FUNCTION_BLOCK FB_LN_IED_LD1_ATCC1 EXTENDS FB_AcsiCommonLogicalNodeClass
VAR_INPUT
	NamPlt: FB_DO_IED_LD1_ATCC1_NamPlt := (sClass:='LPL', bLinkResult:=THIS^.AddDataToContainer(ipData:=NamPlt));
	Beh: FB_DO_IED_LD1_ATCC1_Beh := (sClass:='ENS', bLinkResult:=THIS^.AddDataToContainer(ipData:=Beh));
	Mod_: FB_DO_IED_LD1_ATCC1_Mod := (sObjectName:='Mod', sClass:='ENC', bLinkResult:=THIS^.AddDataToContainer(ipData:=Mod_));
	LocKey: FB_DO_IED_LD1_ATCC1_LocKey := (sClass:='SPS', bLinkResult:=THIS^.AddDataToContainer(ipData:=LocKey));
	CtlV: FB_DO_IED_LD1_ATCC1_CtlV := (sClass:='MV', bLinkResult:=THIS^.AddDataToContainer(ipData:=CtlV));
	TapChg: FB_DO_IED_LD1_ATCC1_TapChg := (sClass:='BSC', bLinkResult:=THIS^.AddDataToContainer(ipData:=TapChg));
	TapPos: FB_DO_IED_LD1_ATCC1_TapPos := (sClass:='ISC', bLinkResult:=THIS^.AddDataToContainer(ipData:=TapPos));
	BndCtrChg: FB_DO_IED_LD1_ATCC1_BndCtrChg := (sClass:='BAC', bLinkResult:=THIS^.AddDataToContainer(ipData:=BndCtrChg));
	ParOp: FB_DO_IED_LD1_ATCC1_ParOp := (sClass:='SPC', bLinkResult:=THIS^.AddDataToContainer(ipData:=ParOp));
END_VAR
VAR
END_VAR

END_FUNCTION_BLOCK
